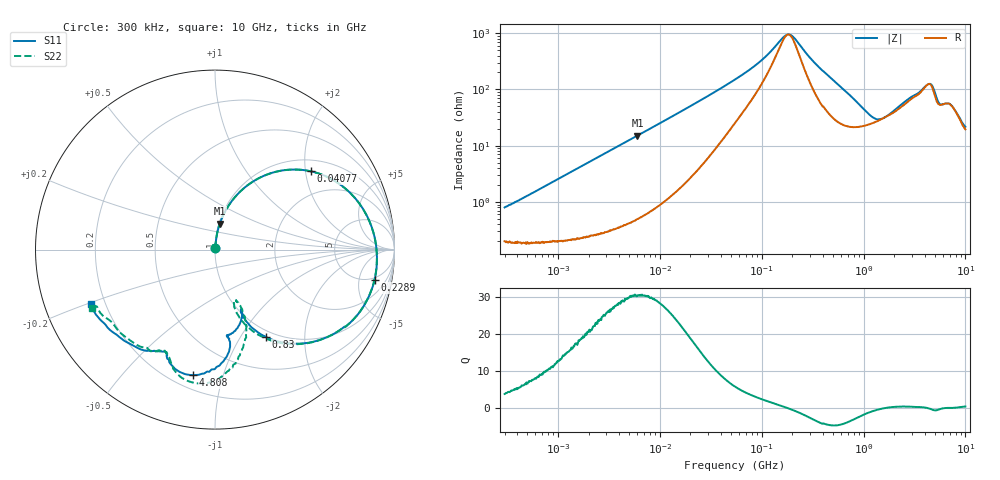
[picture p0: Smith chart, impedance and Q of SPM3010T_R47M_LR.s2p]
! S-Parameter Data Generated by TDK Corporation
! Copyright(C) 2019 TDK Corporation.
! All Rights Reserved.
! TDK P/N: SPM3010T-R47M-LR (Inductor)
! Property: L=470nH at 100kHz
! Size(LxWxT): 3.2x3x1mm
! Model Type: s2p (Touchstone File Format Version 1.0)
! Frequency: DC=Yes Start=0.3MHz Stop=10000MHz 802points Log-sweep
! Model Generated on Sep. 23, 2019
! Port Assignments:
!  1 ---@@@--- 2
! Applicable Conditions:
!  Temperature = 25 degC
!  DC Bias Current = 0 A
!  Small Signal Operation
! Terms and conditions regarding TDK Simulation Models
! (1)This simulation model is being provided solely for informational purposes. Please refer to the specifications of the products in terms of detailed characteristics of such products.
! (2)In no event shall TDK Corporation of any of its subsidiaries be liable for any loss or damage arising, directly or indirectly,
!  From any information contained in this simulation model, including, but not limited to loss or damages arising from any inaccuracies, omissions or errors in connection with such information.
! (3)Any and all copyrights on this simulation model are owned by TDK Corporation.
!  Duplication or redistribution of this simulation model without prior written permission from TDK Corporation is prohibited.
! (4)This simulation model is subject to any modification or change without any prior notice.
! (5)Neither TDK Corporation nor any of its subsidiaries shall make any warranty, express or implied,
!  Including but not limited to the correctness, implied warranties of merchantability and fitness for a particular purpose with respect to this simulation models.
! (6)The use of this simulation model shall be deemed to have consented to the terms and conditions hereof.
# Hz S MA R 50
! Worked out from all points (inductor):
!   801 points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, 300 kHz to 10 GHz, reference 50 ohm
!   read as one part in series: L = 406 nH near 318.3 kHz
!   highest Q = 30.5 at 6.042 MHz (marker M1), where L = 398 nH
!   self-resonance near 181.9 MHz
!   S11 on the Smith chart (normalised r, x): 300 kHz: 1.00, +0.02; 40.77 MHz: 1.29, +2.15; 228.9 MHz: 4.42, -8.27; 830 MHz: 0.91, -1.30; 4.808 GHz: 0.28, -0.80; 10 GHz: 0.15, -0.20
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300000  0.00873 75.3  0.9979 -0.4  0.998 -0.4  0.008383 76.9
1713600  0.04296 84.5  0.9966 -2.5  0.997 -2.5  0.04303 84.6
6041662  0.1476 79.5  0.9839 -8.6  0.9844 -8.6  0.1477 79.5
9671944  0.2315 74.4  0.9645 -13.6  0.9651 -13.6  0.2314 74.4
1.945436e7  0.4293 61.2  0.8808 -25.8  0.8814 -25.8  0.4293 61.2
4.0774e7  0.6909 39.1  0.6472 -44.2  0.6474 -44.2  0.6909 39.1
5.477226e7  0.7717 29.5  0.5183 -50.7  0.5185 -50.7  0.7716 29.5
9.796783e7  0.8672 12.5  0.2723 -55.9  0.2724 -56.0  0.8671 12.4
1.743231e8  0.9035 -2.9  0.09767 -13.1  0.09773 -13.1  0.903 -3.0
2.289088e8  0.905 -10.8  0.1341 36.8  0.1342 36.8  0.9042 -11.0
3.126428e8  0.885 -21.3  0.2603 49.8  0.2604 49.8  0.8834 -21.6
5.285151e8  0.7606 -42.0  0.5147 36.4  0.515 36.4  0.7552 -42.8
8.299813e8  0.5642 -59.7  0.6861 14.0  0.6865 14.0  0.5494 -61.8
1.212691e9  0.4107 -67.2  0.733 -7.3  0.7334 -7.3  0.3784 -71.0
1.767019e9  0.3631 -66.4  0.6878 -29.1  0.6881 -29.1  0.3035 -68.4
2.446702e9  0.4283 -70.7  0.5767 -47.9  0.5769 -47.9  0.3635 -65.5
3.303594e9  0.4814 -81.8  0.4387 -60.0  0.4388 -60.1  0.5456 -72.3
3.991169e9  0.5999 -83.8  0.3455 -67.4  0.3457 -67.4  0.6645 -81.6
4.807583e9  0.7106 -100.0  0.286 -52.2  0.2861 -52.2  0.7513 -97.0
5.849356e9  0.6405 -115.1  0.3746 -64.0  0.3748 -64.1  0.6517 -113.5
7.652089e9  0.7004 -129.6  0.3184 -84.2  0.3183 -84.3  0.6867 -129.4
1e10  0.7555 -156.5  0.2628 -99.7  0.2633 -100.0  0.7594 -154.5
